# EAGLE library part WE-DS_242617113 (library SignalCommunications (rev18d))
WE-DS D-SUB-Filter Connectors Bent 90° Characteristics Standard type filtered with 1000 pF High attenuation of more than 40 dB @ 180 MHz Low size: 6.3 mm Rated voltage: 125 VDC Rated current @ 20 ºC: 5 A Withstand voltage: 250 VRMS Insulation resistance: min. 1000 MΩ Operating temperature: –55 ºC to +125 ºC Applications Filtering of interfaces External connection to -printer -sensor -display Details see: http://katalog.we-online.de/en/pbs/D-SUB-Filter Bent 90° Created on 2015-05-04 2015 (C) Wurth Elektronik
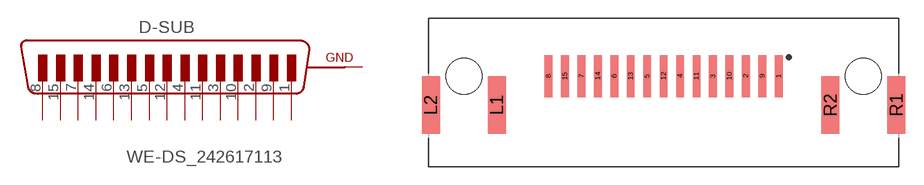
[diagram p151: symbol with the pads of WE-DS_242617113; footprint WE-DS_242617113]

Designator prefix D-SUB

## WE-DS_242617113 (WE-NUMBER: 242617113/15pins_female)  [WE-DS_242617113]
1  8  pas
2  7  pas
3  6  pas
4  5  pas
5  4  pas
6  3  pas
7  2  pas
8  1  pas
9  15  pas
10  14  pas
11  13  pas
12  12  pas
13  11  pas
14  10  pas
15  9  pas
L1  GND  pas
L2  GND  pas
R1  GND  pas
R2  GND  pas

## Footprint WE-DS_242617113 (pad centres in mm)
smd 0.65 x 3.5: 1 9.59,1.37; 2 6.85,1.37; 3 4.11,1.37; 4 1.37,1.37; 5 -1.37,1.37; 6 -4.11,1.37; 7 -6.85,1.37; 8 -9.59,1.37; 9 8.22,1.37; 10 5.48,1.37; 11 2.74,1.37; 12 0,1.37; 13 -2.74,1.37; 14 -5.48,1.37; 15 -8.22,1.37
smd 1.5 x 4.8: L1 -13.9,-1.05; L2 -19.4,-1.05; R1 19.4,-1.05; R2 13.9,-1.05
hole 3 at -16.65,1.35
hole 3 at 16.65,1.35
